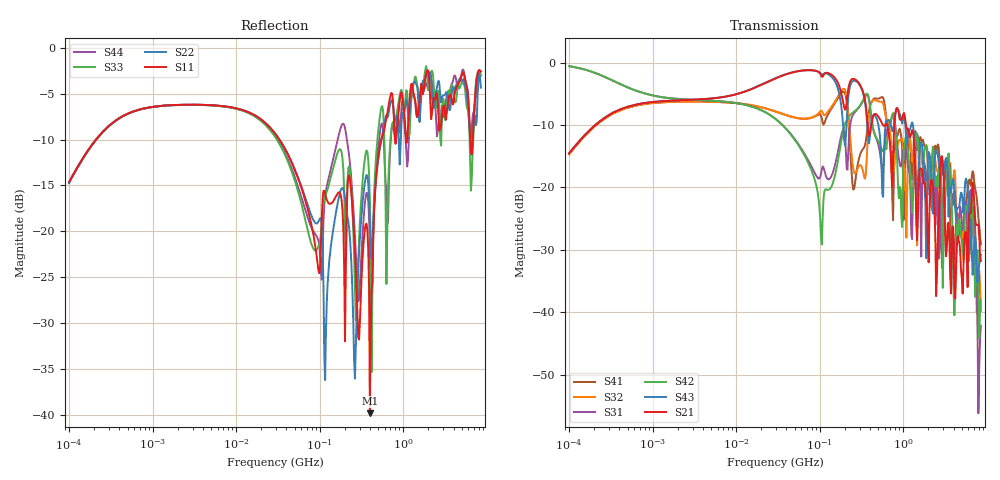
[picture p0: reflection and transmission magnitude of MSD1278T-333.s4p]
# MHz S MA R 50
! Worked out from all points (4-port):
!   498 points, 100 kHz to 8.5 GHz, reference 50 ohm
!   strongest paths, dB at 100 kHz, 1.698 MHz, 29.49 MHz, 500.7 MHz, 8.5 GHz:
!     S21: -14.5, -6.1, -2.5, -8.6, -31.7
!     S43: -14.5, -6.1, -2.5, -9.8, -30.8
!     S42: -0.6, -5.7, -9.0, -12.5, -38.1
!     S31: -0.6, -5.7, -9.0, -13.1, -42.1
!     S32: -14.7, -6.3, -7.8, -6.2, -39.8
!     S41: -14.7, -6.3, -7.8, -5.8, -29.1
!   lowest |S11| = -39.8 dB at 398.4 MHz (marker M1), VSWR 1.02, Z = 50 - j1.02 ohm
!   |S11| at or under -10 dB: 32.89 MHz to 545.9 MHz (513 MHz wide, 177 % of centre); 1.081 GHz to 1.116 GHz (35.39 MHz wide, 3.22 % of centre); 6.344 GHz to 6.801 GHz (456.4 MHz wide, 6.94 % of centre)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
0.1  0.1857 65.9  0.1879 66.8  0.9357 -10.6  0.1846 -113.7
     0.1879 66.8  0.1827 66.5  0.1847 -113.6  0.9363 -10.7
     0.9357 -10.6  0.1847 -113.6  0.1853 66.4  0.1883 66.6
     0.1846 -113.7  0.9363 -10.7  0.1883 66.6  0.1858 66.9
103.5566  0.08549 16.0  0.7927 -28.7  0.1283 -120.0  0.3769 47.4
          0.7927 -28.7  0.1179 -66.6  0.4106 51.3  0.04009 -131.5
          0.1283 -120.0  0.4106 51.3  0.09764 18.4  0.8152 -32.1
          0.3769 47.4  0.04009 -131.5  0.8152 -32.1  0.06003 -5.3
398.4376  0.01018 -87.0  0.2691 -77.9  0.4526 -65.1  0.4488 4.0
          0.2691 -77.9  0.1175 -95.4  0.4248 13.9  0.4595 -60.2
          0.4526 -65.1  0.4248 13.9  0.1455 -73.6  0.2535 -73.2
          0.4488 4.0  0.4595 -60.2  0.2535 -73.2  0.0823 -112.5
2159.325  0.4084 174.0  0.1148 155.6  0.1418 150.5  0.1467 137.1
          0.1148 155.6  0.663 165.1  0.07579 112.3  0.07977 143.0
          0.1418 150.5  0.07579 112.3  0.7429 -179.8  0.1376 78.9
          0.1467 137.1  0.07977 143.0  0.1376 78.9  0.6975 177.4
3651.237  0.5551 13.2  0.01909 0.7  0.08967 -28.4  0.05935 -105.8
          0.01909 0.7  0.4601 3.3  0.1573 -5.3  0.1167 -70.5
          0.08967 -28.4  0.1573 -5.3  0.5128 7.7  0.09991 -60.4
          0.05935 -105.8  0.1167 -70.5  0.09991 -60.4  0.5892 25.8
5898.28  0.5718 -136.5  0.01593 135.4  0.03888 109.4  0.09484 -155.7
         0.01593 135.4  0.4952 -141.7  0.06291 178.6  0.07081 135.5
         0.03888 109.4  0.06291 178.6  0.4607 -126.6  0.09826 -1.3
         0.09484 -155.7  0.07081 135.5  0.09826 -1.3  0.5921 -138.6
8500  0.743 -53.0  0.02586 -101.0  0.007827 -37.4  0.03492 -142.4
      0.02586 -101.0  0.6053 -48.0  0.01028 -159.1  0.0125 -107.9
      0.007827 -37.4  0.01028 -159.1  0.7087 -53.5  0.0289 -39.1
      0.03492 -142.4  0.0125 -107.9  0.0289 -39.1  0.7048 -49.0
